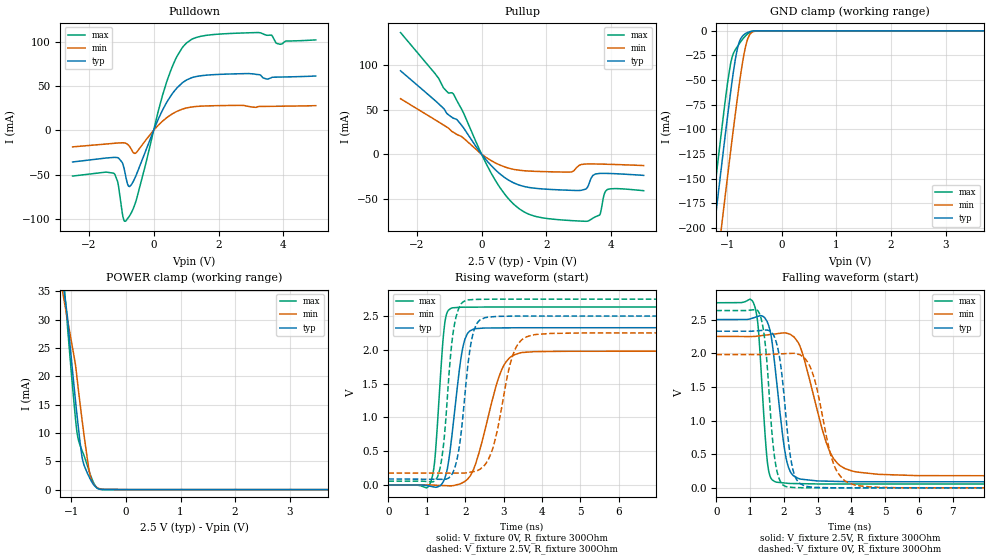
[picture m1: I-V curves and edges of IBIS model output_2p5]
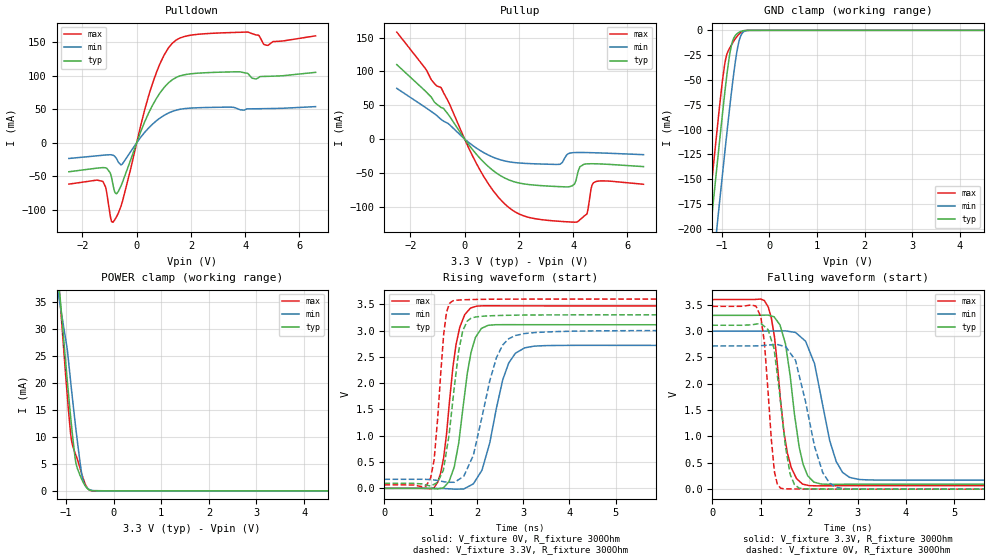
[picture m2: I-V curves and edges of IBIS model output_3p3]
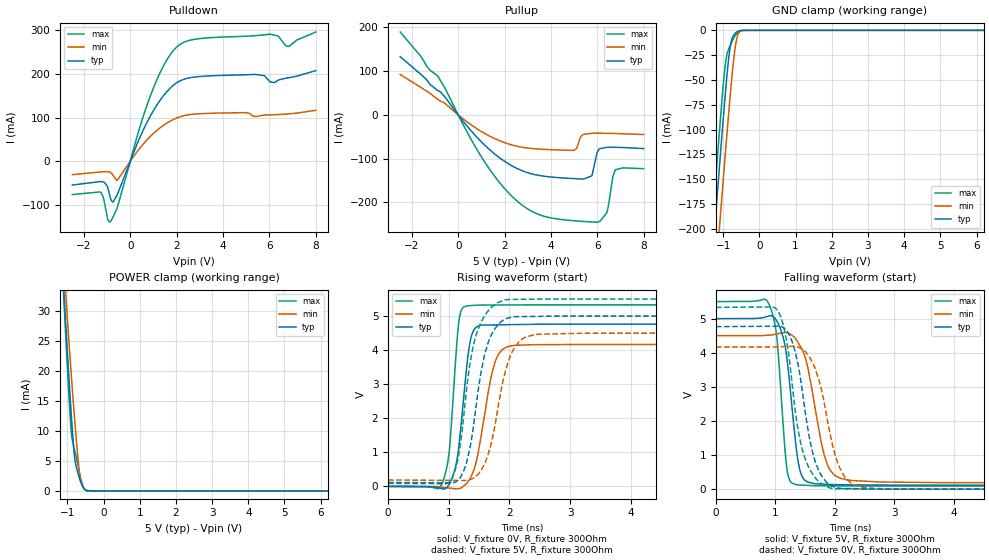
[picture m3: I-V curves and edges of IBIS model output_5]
| TEXAS INSTRUMENTS INCORPORATED
| Standard Linear and Logic Group
| IBIS Model of SN74LV244A-Q1
| OCTAL BUFFER/DRIVER WITH 3-STATE OUTPUTS
| VQFN (WRKS) 20 PIN
[IBIS Ver]   3.2
[Comment Char]  |_char
[File Name]   sn74lv244aq1.ibs
[File_Rev]   0.0
[Date]   Aug, 4, 2022
[Source]   Data created from simulations
[Notes]   The following is an IBIS list for the LV244A.
|   The warning about non-monotonic V-I curves might be reported,
|   but it is NAo ampere region and negligible.
|   The warning about AC Rising Endpoint might be reported,
|   but it is due to HSPICE issue and negligible.
[Disclaimer] Property of Texas Instruments Incorporated.  Unauthorized
   reproduction and/or distribution is strictly prohibited.
   This product is protected under copyright law.
   Created 2022, (C) Copyright 2022, Texas Instruments Inc.,
   All Rights Reserved.
   UNLESS THERE IS A SIGNED, WRITTEN AGREEMENT TO THE
   CONTRARY, TEXAS INSTRUMENTS ("TI") IS PROVIDING THE IBIS
   MODELS "AS IS" AND WITHOUT ANY WARRANTY, EXPRESSED OR
   IMPLIED.  TI assumes no liability for:
   1) the accuracy of the IBIS models provided to your
   company;
   2) the proper functioning of these IBIS Models in your
   design or for any resulting applications; or
   3) infringement of patents, copyrights or intellectual
   property rights resulting from your use of these IBIS
   models.
   TI provides IBIS Models as a service to our customers.
   You and your company shall not distribute, sell or give
   these models to anyone else without prior written
   permission from TI.
   TI reserves the right to make changes to our products or
   to discontinue any semiconductor product or service
   without notice, and advises our customers to obtain the
   latest version of relevant information to verify, before
   placing orders, that the information being relied on is
   current.
   Please be aware that your receipt and use of the IBIS
   information provided shall serve as acceptance of these
   terms and conditions.  If you do not accept these terms,
   you should return or destroy the IBIS models and any
   other accompanying information immediately.
|   Device
[Component]   SN74LV244A_WRKS
[Manufacturer]   TI
[Package]   |VQFN, 20 pin RKS
|   typ   min   max
R_pkg   0.0928   0.0773   0.1056
L_pkg   1.6543nH   1.401nH   1.9974nH
C_pkg   0.2150pF   0.1865pF   0.2577pF
[Pin]   signal_name   model_name   R_pin   L_pin   C_pin
1   1OE/   GND   NA   NA   NA
2   1A1   INPUT   NA   NA   NA
3   2Y4   OUTPUT   NA   NA   NA
4   1A2   INPUT   NA   NA   NA
5   2Y3   OUTPUT   NA   NA   NA
6   1A3   INPUT   NA   NA   NA
7   2Y2   OUTPUT   NA   NA   NA
8   1A4   INPUT   NA   NA   NA
9   2Y1   OUTPUT   NA   NA   NA
10   GND   GND   NA   NA   NA
11   2A1   INPUT   NA   NA   NA
12   1Y4   OUTPUT   NA   NA   NA
13   2A2   INPUT   NA   NA   NA
14   1Y3   OUTPUT   NA   NA   NA
15   2A3   INPUT   NA   NA   NA
16   1Y2   OUTPUT   NA   NA   NA
17   2A4   INPUT   NA   NA   NA
18   1Y1   OUTPUT   NA   NA   NA
19   2OE/   INPUT   NA   NA   NA
20   VCC   POWER   NA   NA   NA
[Model Selector]   INPUT
input_2p5   2.5-V Vcc Input Model
input_3p3   3.3-V Vcc Input Model
input_5   5.0-V Vcc Input Model
[Model Selector]   OUTPUT
output_2p5   2.5-V Vcc Output Model
output_3p3   3.3-V Vcc Output Model
output_5   5.0-V Vcc Output Model
| Models and submodels in the file (6): output_2p5 (Output), output_3p3 (Output), output_5 (Output), input_2p5 (Input), input_3p3 (Input), input_5 (Input)
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[Model]   output_2p5
Model_type   Output
Polarity   Non-Inverting
Vmeas = 0.9
Vref = 0.9
Cref = 15pF
Rref = 100000
|   typ   min   max
C_comp   4.947pF   4.835pF   5.043pF
[Voltage Range]   2.5   2.25   2.75
[Temperature Range]   27   125   -40
[Pullup Reference]   2.5   2.25   2.75
[Pulldown Reference]   -0   0   0
[Power Clamp Reference]   2.5   2.25   2.75
[GND Clamp Reference]   0   0   0
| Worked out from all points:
|   slope of the pulldown table from 0 to 0.375 V, typ, clamps not added: 12.6 ohm
|   slope of the pullup table from 0 to 0.375 V, typ, clamps not added: 24 ohm
|   GND clamp passes 1 mA (typ) near -0.59 V on its own axis
|   POWER clamp passes 1 mA (typ) near -0.60 V on its own axis
|   falling waveform, V_fixture 2.5V, R_fixture 300Ohm: 20-80 % time 335ps typ, 676ps min, 207ps max; typ from 2.5 V to 0.088 V
|   rising waveform, V_fixture 0V, R_fixture 300Ohm: 20-80 % time 290ps typ, 552ps min, 186ps max; typ from 0 V to 2.33 V
|   rising waveform, V_fixture 2.5V, R_fixture 300Ohm: 20-80 % time 280ps typ, 452ps min, 240ps max; typ from 0.088 V to 2.5 V
|   falling waveform, V_fixture 0V, R_fixture 300Ohm: 20-80 % time 298ps typ, 523ps min, 252ps max; typ from 2.33 V to 0 V
[Pulldown]
|   Voltage   I(typ)   I(min)   I(max)
-2.5V     -35.79mA   -18.74mA   -51.7mA
-1.23V    -30.63mA   -14.75mA   -48.54mA
-1.114V   -30.88mA   -14.41mA   -57.55mA
-956.5mV  -37.5mA    -14.14mA   -95.94mA
-872.5mV  -50.05mA   -14.51mA   -102.7mA
-683.5mV  -61.25mA   -21.9mA    -92.7mA
-536.5mV  -50.33mA   -25.2mA    -78.68mA
387.5mV   30.58mA    13.77mA    53.11mA
1.018V    56.81mA    25.22mA    98.68mA
3.159V    63.05mA    25.84mA    110.2mA
3.894V    60.03mA    27.12mA    97.09mA
4.997V    61.2mA     27.76mA    102mA
[GND Clamp]
|   Voltage   I(typ)   I(min)   I(max)
-2.5V     -817.8mA   -872.3mA   -789.1mA
-1.303V   -231.2mA   -292.1mA   -196.1mA
-1.23V    -196.2mA   -257.3mA   -160.8mA
-1.125V   -146.7mA   -208.1mA   -111.2mA
-1.062V   -117.5mA   -178.9mA   -82.22mA
-946mV    -65.86mA   -126.2mA   -35.86mA
-830.5mV  -22.76mA   -75.49mA   -17.36mA
-767.5mV  -9.785mA   -49.8mA    -12.22mA
-694mV    -3.965mA   -24.23mA   -6.893mA
-589mV    -891.1uA   -3.999mA   -1.764mA
-431.5mV  -12.85uA   -82.5uA    -10.97uA
8V        0A         0A         0A
[Pullup]
|   Voltage   I(typ)   I(min)   I(max)
-2.5V     93.52mA    62.21mA    136.3mA
-1.177V   51.48mA    32.8mA     74.46mA
-872.5mV  40.36mA    24.61mA    67.72mA
282.5mV   -12.23mA   -6.873mA   -20.4mA
1.165V    -34.63mA   -17.96mA   -61.26mA
2.75V     -40.43mA   -19.9mA    -74.3mA
3.275V    -36.4mA    -10.9mA    -74.93mA
3.433V    -23.71mA   -10.89mA   -71.59mA
3.643V    -21.51mA   -11.02mA   -68.06mA
3.779V    -21.44mA   -11.14mA   -45.04mA
3.873V    -21.49mA   -11.24mA   -39.63mA
4.997V    -23.68mA   -12.67mA   -40.87mA
[POWER Clamp]
|   Voltage   I(typ)   I(min)   I(max)
-2.5V     142.8mA    115.5mA    175.3mA
-1.167V   37.39mA    35.21mA    40.36mA
-1.083V   31.33mA    30.63mA    30.15mA
-935.5mV  16.74mA    22.66mA    13.62mA
-904mV    13.8mA     20.34mA    10.62mA
-883mV    11.92mA    18.58mA    9.292mA
-799mV    5.487mA    11.92mA    6.762mA
-757mV    4.04mA     8.831mA    5.712mA
-662.5mV  2.013mA    2.787mA    2.926mA
-589mV    837.6uA    921.3uA    1.128mA
-494.5mV  114.2uA    194.6uA    87.23uA
8V        0A         0A         0A
[Ramp]
R_load = 300
|   typ   min   max
dV/dt_r   1.39637/2.89983e-10   1.18808/5.507e-10   1.58042/1.85495e-10
dV/dt_f   1.44698/3.33617e-10   1.24493/6.73372e-10   1.61611/2.0617e-10
[Falling Waveform]
V_fixture = 2.5V
V_fixture_min = 2.25V
V_fixture_max = 2.75V
R_fixture = 300Ohm
C_fixture = 0F
|   Time   V(typ)   V(min)   V(max)
0s        2.5V       2.25V      2.75V
1.136ns   2.531V     2.249V     2.703V
1.249ns   2.549V     2.256V     2.348V
1.522ns   2.452V     2.273V     353.9mV
1.741ns   1.797V     2.287V     91.27mV
2.018ns   588.3mV    2.302V     72.43mV
2.221ns   216.9mV    2.27V      64.78mV
3.34ns    98.56mV    564.5mV    57.79mV
4.014ns   91.09mV    251.9mV    57.71mV
15ns      88.36mV    175.1mV    56.48mV
[Rising Waveform]
V_fixture = 0V
V_fixture_min = 0V
V_fixture_max = 0V
R_fixture = 300Ohm
C_fixture = 0F
|   Time   V(typ)   V(min)   V(max)
0s        3.396uV    3.144uV    3.15uV
1.101ns   -20.53mV   -1.038mV   39.04mV
1.22ns    -33.89mV   -3.902mV   434.5mV
1.451ns   73.9mV     -9.484mV   2.309V
1.638ns   651.2mV    -13.49mV   2.616V
1.875ns   1.814V     16.57mV    2.63V
2.052ns   2.233V     80.31mV    2.631V
2.947ns   2.324V     1.699V     2.633V
3.415ns   2.326V     1.953V     2.633V
15ns      2.327V     1.98V      2.634V
[Rising Waveform]
V_fixture = 2.5V
V_fixture_min = 2.25V
V_fixture_max = 2.75V
R_fixture = 300Ohm
C_fixture = 0F
|   Time   V(typ)   V(min)   V(max)
0s        88.36mV    175.1mV    56.48mV
1.276ns   83.48mV    175.3mV    113.8mV
1.434ns   82.88mV    175.4mV    581.9mV
1.697ns   205.1mV    175.4mV    2.292V
2.014ns   1.459V     177.7mV    2.731V
2.347ns   2.421V     220.4mV    2.747V
2.726ns   2.49V      553mV      2.749V
3.249ns   2.498V     1.934V     2.75V
3.735ns   2.5V       2.216V     2.75V
15ns      2.5V       2.25V      2.75V
[Falling Waveform]
|Gnd
V_fixture = 0V
V_fixture_min = 0V
V_fixture_max = 0V
R_fixture = 300Ohm
C_fixture = 0F
|   Time   V(typ)   V(min)   V(max)
0s        2.327V     1.98V      2.634V
1.286ns   2.336V     1.98V      2.584V
1.467ns   2.344V     1.98V      2.058V
1.741ns   2.219V     1.987V     404.8mV
2.048ns   1.149V     1.994V     21.5mV
2.428ns   88.13mV    1.984V     3.239mV
2.902ns   8.09mV     1.628V     404.1uV
3.534ns   601.5uV    284.6mV    383.2uV
4.074ns   573.4uV    46.92mV    365.3uV
15ns      3.396uV    3.144uV    3.15uV
[Model]   output_3p3
Model_type   Output
Polarity   Non-Inverting
Vmeas = 1.5
Vref = 0
Cref = 15pF
Rref = 1000000
|   typ   min   max
C_comp   4.947pF   4.835pF   5.043pF
[Voltage Range]   3.3   3   3.6
[Temperature Range]   27   125   -40
[Pullup Reference]   3.3   3   3.6
[Pulldown Reference]   0   0   0
[Power Clamp Reference]   3.3   3   3.6
[GND Clamp Reference]   0   0   0
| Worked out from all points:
|   slope of the pulldown table from 0 to 0.495 V, typ, clamps not added: 10.1 ohm
|   slope of the pullup table from 0 to 0.495 V, typ, clamps not added: 19.6 ohm
|   GND clamp passes 1 mA (typ) near -0.59 V on its own axis
|   POWER clamp passes 1 mA (typ) near -0.60 V on its own axis
|   falling waveform, V_fixture 3.3V, R_fixture 300Ohm: 20-80 % time 283ps typ, 398ps min, 251ps max; typ from 3.3 V to 0.094 V
|   rising waveform, V_fixture 0V, R_fixture 300Ohm: 20-80 % time 298ps typ, 430ps min, 263ps max; typ from 0 V to 3.11 V
|   rising waveform, V_fixture 3.3V, R_fixture 300Ohm: 20-80 % time 269ps typ, 455ps min, 181ps max; typ from 0.094 V to 3.3 V
|   falling waveform, V_fixture 0V, R_fixture 300Ohm: 20-80 % time 245ps typ, 413ps min, 168ps max; typ from 3.11 V to 0 V
[Pulldown]
|   Voltage   I(typ)   I(min)   I(max)
-2.5V     -43.18mA   -23.37mA   -61.62mA
-1.25V    -37.01mA   -18.58mA   -57.53mA
-977.5mV  -44.66mA   -17.83mA   -108.2mA
-851.5mV  -66.87mA   -18.96mA   -117.3mA
-746.5mV  -76.02mA   -23.35mA   -110.5mA
-547mV    -61.15mA   -32.26mA   -90.4mA
576.5mV   55.38mA    27.5mA     87.6mA
1.018V    82.74mA    41.05mA    131.3mA
1.49V     98.08mA    49.01mA    154mA
4.104V    103mA      50.58mA    165mA
4.84V     99.09mA    50.98mA    145.2mA
6.593V    105mA      53.91mA    159.4mA
[GND Clamp]
|   Voltage   I(typ)   I(min)   I(max)
-2.5V     -817.8mA   -872.3mA   -789.1mA
-1.303V   -231.2mA   -292.1mA   -196.1mA
-1.23V    -196.2mA   -257.3mA   -160.8mA
-1.125V   -146.7mA   -208.1mA   -111.2mA
-1.062V   -117.5mA   -178.9mA   -82.22mA
-946mV    -65.86mA   -126.2mA   -35.86mA
-830.5mV  -22.76mA   -75.49mA   -17.36mA
-767.5mV  -9.785mA   -49.8mA    -12.22mA
-694mV    -3.965mA   -24.23mA   -6.893mA
-589mV    -891.1uA   -3.999mA   -1.764mA
-431.5mV  -12.85uA   -82.5uA    -10.97uA
8V        0A         0A         0A
[Pullup]
|   Voltage   I(typ)   I(min)   I(max)
-2.5V     110mA      74.9mA     158.1mA
-872.5mV  46.71mA    29.17mA    76.33mA
702.5mV   -34.17mA   -20.06mA   -55.22mA
1.805V    -62.92mA   -34.63mA   -106.3mA
3.495V    -70.37mA   -37.38mA   -121.6mA
3.968V    -69.17mA   -20.26mA   -122.8mA
4.115V    -59.51mA   -19.94mA   -122.8mA
4.252V    -40.97mA   -19.89mA   -119.3mA
4.503V    -36.74mA   -20.02mA   -111mA
4.661V    -36.53mA   -20.17mA   -73.41mA
4.745V    -36.55mA   -20.26mA   -64.8mA
6.593V    -40.77mA   -23.12mA   -66.88mA
[POWER Clamp]
|   Voltage   I(typ)   I(min)   I(max)
-2.5V     144.5mA    117mA      177mA
-1.219V   42.82mA    39.69mA    46.86mA
-1.125V   35.89mA    34.5mA     35.22mA
-977.5mV  20.83mA    26.44mA    18.04mA
-914.5mV  14.77mA    21.23mA    11.56mA
-883mV    11.92mA    18.58mA    9.292mA
-799mV    5.487mA    11.92mA    6.762mA
-715mV    3.079mA    5.916mA    4.489mA
-662.5mV  2.013mA    2.787mA    2.926mA
-589mV    837.6uA    921.4uA    1.128mA
-494.5mV  114.2uA    194.6uA    87.23uA
8V        0A         0A         0A
[Ramp]
R_load = 300
|   typ   min   max
dV/dt_r   1.86701/2.97801e-10   1.63117/4.29678e-10   2.08197/2.62916e-10
dV/dt_f   1.92339/2.82985e-10   1.69703/3.98282e-10   2.12049/2.514e-10
[Falling Waveform]
V_fixture = 3.3V
V_fixture_min = 3V
V_fixture_max = 3.6V
R_fixture = 300Ohm
C_fixture = 0F
|   Time   V(typ)   V(min)   V(max)
0s        3.3V       3V         3.6V
1.154ns   3.303V     3.001V     3.457V
1.282ns   3.263V     3.003V     2.899V
1.481ns   2.851V     3.004V     1.073V
1.548ns   2.521V     2.999V     692.6mV
1.863ns   517.6mV    2.859V     95.81mV
2.11ns    130.4mV    2.382V     64.36mV
2.559ns   93.23mV    522mV      64.97mV
2.834ns   93.79mV    223.6mV    65.5mV
15ns      94.34mV    171.6mV    65.84mV
[Rising Waveform]
V_fixture = 0V
V_fixture_min = 0V
V_fixture_max = 0V
R_fixture = 300Ohm
C_fixture = 0F
|   Time   V(typ)   V(min)   V(max)
0s        954.7nV    1.301uV    430.7nV
1.075ns   -7.226mV   24.91uV    13.43mV
1.282ns   14.79mV    -4.189mV   590.9mV
1.397ns   128.6mV    -8.874mV   1.554V
1.628ns   1.017V     -13.82mV   3.059V
1.793ns   2.191V     23.38mV    3.36V
2ns       2.912V     191.2mV    3.467V
2.689ns   3.113V     2.384V     3.471V
3.034ns   3.113V     2.672V     3.47V
15ns      3.112V     2.719V     3.47V
[Rising Waveform]
V_fixture = 3.3V
V_fixture_min = 3V
V_fixture_max = 3.6V
R_fixture = 300Ohm
C_fixture = 0F
|   Time   V(typ)   V(min)   V(max)
0s        94.34mV    171.6mV    65.84mV
1ns       43.1mV     166.4mV    202mV
1.075ns   77.89mV    157.9mV    541.9mV
1.282ns   382.8mV    127.1mV    2.935V
1.481ns   1.681V     115.3mV    3.567V
1.608ns   2.623V     167.7mV    3.581V
1.793ns   3.183V     377.2mV    3.589V
2.424ns   3.286V     2.487V     3.598V
2.834ns   3.294V     2.908V     3.599V
15ns      3.3V       3V         3.6V
[Falling Waveform]
|Gnd
V_fixture = 0V
V_fixture_min = 0V
V_fixture_max = 0V
R_fixture = 300Ohm
C_fixture = 0F
|   Time   V(typ)   V(min)   V(max)
0s        3.112V     2.719V     3.47V
1ns       3.147V     2.724V     3.276V
1.075ns   3.088V     2.729V     2.786V
1.282ns   2.614V     2.743V     329.4mV
1.409ns   1.649V     2.73V      17.99mV
1.51ns    803mV      2.703V     4.982mV
1.695ns   85.9mV     2.473V     3.495mV
2.279ns   3.002mV    314.4mV    1.041mV
2.559ns   1.781mV    36.9mV     569.7uV
15ns      463nV      1.302uV    432.5nV
[Model]   output_5
Model_type   Output
Polarity   Non-Inverting
Vmeas = 1.5
Vref = 0.9
Cref = 15pF
Rref = 100000
|   typ   min   max
C_comp   4.947pF   4.835pF   5.043pF
[Voltage Range]   5   4.5   5.5
[Temperature Range]   27   125   -40
[Pullup Reference]   5   4.5   5.5
[Pulldown Reference]   -0   0   0
[Power Clamp Reference]   5   4.5   5.5
[GND Clamp Reference]   0   0   0
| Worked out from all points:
|   slope of the pulldown table from 0 to 0.75 V, typ, clamps not added: 8.16 ohm
|   slope of the pullup table from 0 to 0.75 V, typ, clamps not added: 15.7 ohm
|   GND clamp passes 1 mA (typ) near -0.59 V on its own axis
|   POWER clamp passes 1 mA (typ) near -0.60 V on its own axis
|   falling waveform, V_fixture 5V, R_fixture 300Ohm: 20-80 % time 179ps typ, 278ps min, 134ps max; typ from 5 V to 0.116 V
|   rising waveform, V_fixture 0V, R_fixture 300Ohm: 20-80 % time 164ps typ, 247ps min, 125ps max; typ from 0 V to 4.76 V
|   rising waveform, V_fixture 5V, R_fixture 300Ohm: 20-80 % time 271ps typ, 311ps min, 262ps max; typ from 0.116 V to 5 V
|   falling waveform, V_fixture 0V, R_fixture 300Ohm: 20-80 % time 284ps typ, 331ps min, 272ps max; typ from 4.76 V to 0 V
[Pulldown]
|   Voltage   I(typ)   I(min)   I(max)
-2.5V     -54.17mA   -30.47mA   -76mA
-1.292V   -46.43mA   -24.52mA   -69.97mA
-998.5mV  -56.07mA   -23.49mA   -125.9mA
-872.5mV  -81.07mA   -24.92mA   -138.7mA
-757mV    -93.39mA   -30.82mA   -128.9mA
-547mV    -74.32mA   -42.13mA   -103.1mA
1.018V    117.6mA    64.62mA    170mA
2.162V    184.3mA    102.1mA    268mA
5.407V    198.7mA    102.2mA    287.3mA
6.026V    181.7mA    106.1mA    290.8mA
6.845V    191.1mA    108.5mA    262.7mA
8V        207.3mA    116.6mA    295.4mA
[GND Clamp]
|   Voltage   I(typ)   I(min)   I(max)
-2.5V     -817.8mA   -872.3mA   -789.1mA
-1.303V   -231.2mA   -292.1mA   -196.1mA
-1.23V    -196.2mA   -257.3mA   -160.8mA
-1.125V   -146.7mA   -208.1mA   -111.2mA
-1.062V   -117.5mA   -178.9mA   -82.22mA
-946mV    -65.86mA   -126.2mA   -35.86mA
-830.5mV  -22.76mA   -75.49mA   -17.36mA
-767.5mV  -9.785mA   -49.8mA    -12.22mA
-694mV    -3.965mA   -24.23mA   -6.893mA
-589mV    -891.1uA   -3.999mA   -1.764mA
-431.5mV  -12.85uA   -82.5uA    -10.98uA
8V        0A         0A         0A
[Pullup]
|   Voltage   I(typ)   I(min)   I(max)
-2.5V     133.2mA    92.38mA    189.5mA
-872.5mV  55.54mA    35.32mA    88.38mA
1.532V    -87.54mA   -53.13mA   -137.5mA
3.149V    -134.5mA   -76.7mA    -219.8mA
5.018V    -145.8mA   -80.62mA   -242.3mA
5.407V    -146.7mA   -44.46mA   -243.8mA
5.763V    -139.4mA   -41.98mA   -244.9mA
6.058V    -79.55mA   -41.85mA   -244.8mA
6.415V    -74.24mA   -42.14mA   -223.5mA
6.667V    -74mA      -42.47mA   -142.1mA
6.771V    -74.07mA   -42.63mA   -126.1mA
8V        -77.02mA   -44.9mA    -123mA
[POWER Clamp]
|   Voltage   I(typ)   I(min)   I(max)
-2.5V     147.9mA    120.2mA    180.7mA
-1.177V   41.53mA    40.53mA    41.66mA
-1.072V   30.45mA    34.72mA    28.9mA
-1.04V    27.19mA    32.3mA     25.19mA
-946mV    17.75mA    23.94mA    14.69mA
-893.5mV  12.85mA    19.46mA    9.879mA
-799mV    5.488mA    11.92mA    6.762mA
-725.5mV  3.307mA    6.625mA    4.806mA
-652mV    1.818mA    2.364mA    2.632mA
-589mV    837.6uA    921.4uA    1.128mA
-494.5mV  114.2uA    194.6uA    87.23uA
8V        0A         0A         0A
[Ramp]
R_load = 300
|   typ   min   max
dV/dt_r   2.85909/1.64227e-10   2.50123/2.46513e-10   3.1981/1.25452e-10
dV/dt_f   2.93049/1.78709e-10   2.58732/2.77607e-10   3.24613/1.34209e-10
[Falling Waveform]
V_fixture = 5V
V_fixture_min = 4.5V
V_fixture_max = 5.5V
R_fixture = 300Ohm
C_fixture = 0F
|   Time   V(typ)   V(min)   V(max)
0s        5V         4.5V       5.5V
899.3ps   5.081V     4.518V     5.399V
1.027ns   4.927V     4.552V     4.401V
1.158ns   4.241V     4.593V     1.212V
1.221ns   3.406V     4.569V     344.8mV
1.351ns   1.197V     4.381V     132.3mV
1.482ns   281.8mV    3.954V     115.5mV
1.867ns   144.1mV    750.4mV    97.94mV
2.206ns   127.4mV    272.9mV    94.17mV
15ns      115.8mV    187.8mV    89.78mV
[Rising Waveform]
V_fixture = 0V
V_fixture_min = 0V
V_fixture_max = 0V
R_fixture = 300Ohm
C_fixture = 0F
|   Time   V(typ)   V(min)   V(max)
0s        1.427uV    1.371uV    1.299uV
889.8ps   -68.08mV   -22.9mV    87.87mV
1.008ns   60.88mV    -47.63mV   1.036V
1.131ns   733mV      -73.02mV   4.163V
1.196ns   1.681V     -48.48mV   5.116V
1.304ns   3.643V     105mV      5.301V
1.426ns   4.628V     553.3mV    5.315V
1.754ns   4.742V     3.607V     5.325V
2.032ns   4.749V     4.128V     5.327V
15ns      4.765V     4.169V     5.33V
[Rising Waveform]
V_fixture = 5V
V_fixture_min = 4.5V
V_fixture_max = 5.5V
R_fixture = 300Ohm
C_fixture = 0F
|   Time   V(typ)   V(min)   V(max)
0s        115.8mV    187.8mV    89.78mV
995.3ps   103mV      178.1mV    107.5mV
1.184ns   245.3mV    176.3mV    1.154V
1.339ns   1.054V     197.9mV    3.493V
1.456ns   2.432V     311.6mV    4.468V
1.646ns   4.203V     924.2mV    5.145V
1.926ns   4.908V     3.332V     5.475V
2.163ns   4.985V     4.258V     5.493V
2.456ns   4.992V     4.466V     5.498V
15ns      5V         4.5V       5.5V
[Falling Waveform]
|Gnd
V_fixture = 0V
V_fixture_min = 0V
V_fixture_max = 0V
R_fixture = 300Ohm
C_fixture = 0F
|   Time   V(typ)   V(min)   V(max)
0s        4.765V     4.169V     5.33V
1.043ns   4.78V      4.174V     5.225V
1.186ns   4.655V     4.184V     4.369V
1.288ns   4.292V     4.191V     2.977V
1.481ns   2.51V      4.059V     989.1mV
1.671ns   798mV      3.519V     330.4mV
1.926ns   115.5mV    1.563V     29.66mV
2.163ns   20.64mV    368.4mV    9.044mV
2.571ns   7.108mV    32.68mV    429.2uV
15ns      1.427uV    1.371uV    1.299uV
